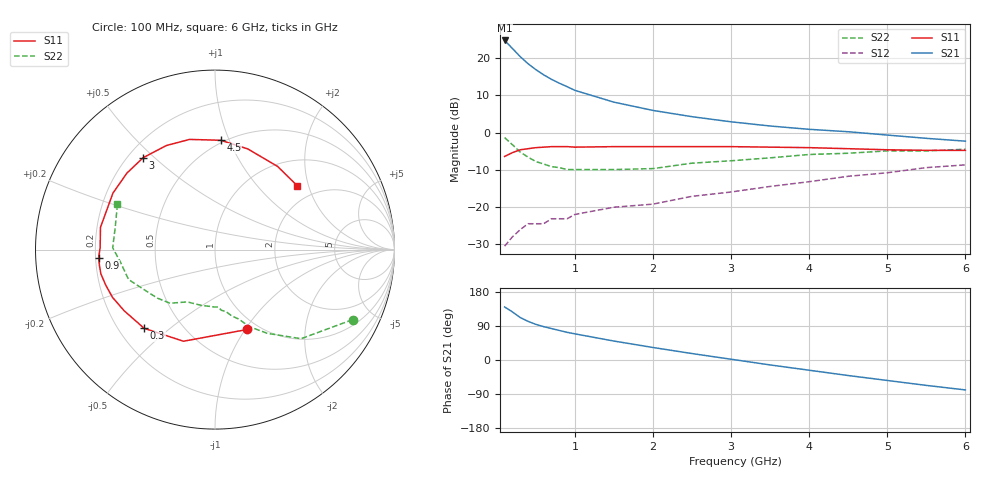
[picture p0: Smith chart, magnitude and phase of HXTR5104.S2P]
! HXTR-5104 Common Emitter
! Vce=18V  Ic=110mA
# ghz s ma r 50
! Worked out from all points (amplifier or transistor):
!   20 points, 100 MHz to 6 GHz, reference 50 ohm
!   highest |S21| = 24.8 dB at 100 MHz (marker M1)
!   |S21| within 3 dB of that: start of sweep to 238.7 MHz
!   unconditionally stable (mu >= 1): 1.702 GHz to 2.386 GHz
!   at 400 MHz: K = 0.45, MSG = 21.5 dB, |S12| = -24.4 dB
!   at 1.5 GHz: K = 0.94, MSG = 14.1 dB, |S12| = -20.0 dB
!   at 6 GHz: K = 0.70, MSG = 3.2 dB, |S12| = -8.6 dB
!   S11 on the Smith chart (normalised r, x): 100 MHz: 0.88, -1.02; 300 MHz: 0.30, -0.41; 900 MHz: 0.21, -0.03; 3 GHz: 0.26, +0.46; 4.5 GHz: 0.48, +0.93; 6 GHz: 1.57, +1.69
0.1  0.48 -68.0  17.3 140.0  0.03 62.0  0.86 -27.0
0.2  0.54 -109.0  13.5 127.0  0.04 48.0  0.69 -46.0
0.3  0.59 -132.0  10.5 112.0  0.05 40.0  0.55 -58.0
0.4  0.61 -146.0  8.43 102.0  0.06 36.0  0.47 -66.0
0.5  0.63 -155.0  7.02 94.0  0.06 34.0  0.41 -71.0
0.6  0.64 -162.0  5.98 88.0  0.06 33.0  0.38 -76.0
0.7  0.65 -168.0  5.21 83.0  0.07 33.0  0.35 -80.0
0.8  0.65 -172.0  4.62 78.0  0.07 33.0  0.34 -84.0
0.9  0.65 -176.0  4.15 73.0  0.07 33.0  0.32 -87.0
1  0.64 179.0  3.7 69.0  0.08 32.0  0.32 -90.0
1.5  0.65 169.0  2.57 50.0  0.1 31.0  0.32 -104.0
2  0.65 151.0  1.99 33.0  0.11 30.0  0.33 -118.0
2.5  0.65 139.0  1.64 17.0  0.14 25.0  0.39 -130.0
3  0.65 128.0  1.4 2.0  0.16 20.0  0.42 -140.0
3.5  0.64 115.0  1.23 -13.0  0.19 14.0  0.46 -152.0
4  0.63 103.0  1.11 -27.0  0.22 5.0  0.51 -161.0
4.5  0.61 87.0  1.03 -41.0  0.26 -2.0  0.53 -172.0
5  0.59 72.0  0.93 -54.0  0.29 -12.0  0.57 179.0
5.5  0.58 53.0  0.84 -67.0  0.34 -22.0  0.57 167.0
6  0.58 38.0  0.77 -79.0  0.37 -31.0  0.6 155.0
